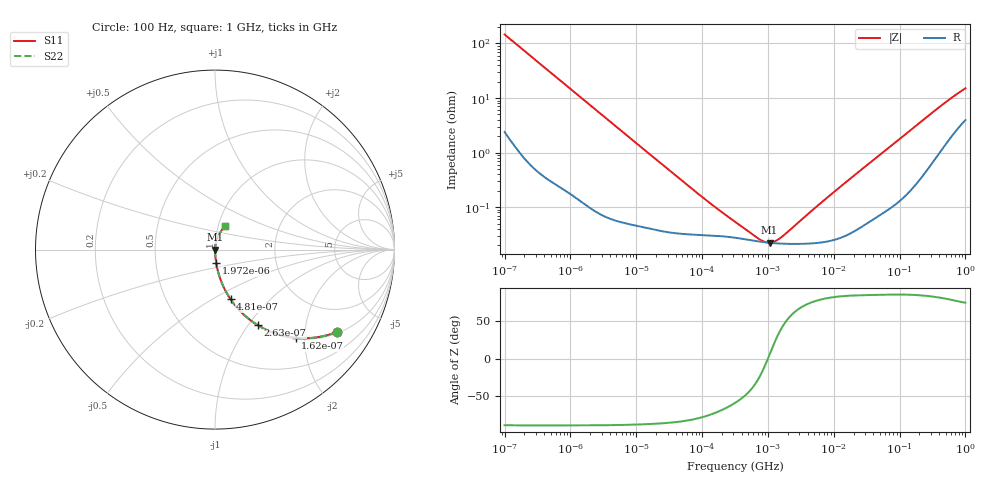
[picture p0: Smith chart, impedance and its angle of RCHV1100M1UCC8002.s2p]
! RCHV1100M1UCC8002  S-PARAMETER MODEL  (AEC-Q200 qualified)
! Model Generated by ELNA Corporation (http://www.ty-top.com)
! Version 1.0
! ELNA Control No. 240229
! Copyright (c) 2024 ELNA CO.,LTD. All Rights Reserved.
! Products Name : CONDUCTIVE POLYMER HYBRID ALUMINUM ELECTROLYTIC CAPACITORS
! Characteristics :
!  Capacitance  :  10uF  ,  Rated voltage  :  50V
!  Operating Temp. Range  :  -55 to +105 degC  ,  Endurance  :  5000hr at 105 degC
!  Dimension D  :  5mm  ,  Dimension L  :  5.8mm
! Frequency Range : 100Hz - 1GHz
! External Node Assignments :
!  1  o---| |---o  2
# MHz S RI R 50
!Freq[MHz].  S11 Real  S11 Imag  S21 Real  S21 Imag  S12 Real  S12 Imag  S22 Real  S22 Imag
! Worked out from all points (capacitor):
!   401 points, 100 Hz to 1 GHz, reference 50 ohm
!   read as one part in series: C = 10.9 uF near 108 Hz
!   lowest |Z| = 22.4 mohm at 1.059 MHz (marker M1)
!   series resonance near 1 MHz, so ESL is about 2.3 nH
!   S11 on the Smith chart (normalised r, x): 100 Hz: 1.05, -2.92; 162 Hz: 1.02, -1.80; 263 Hz: 1.01, -1.11; 481 Hz: 1.01, -0.61; 1.972 kHz: 1.00, -0.15; 1 GHz: 1.08, +0.29
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0.0001  0.6781 -0.4591  0.3219 0.4591  0.3219 0.4591  0.6781 -0.4591
0.000162  0.4485 -0.4915  0.5515 0.4915  0.5515 0.4915  0.4485 -0.4915
0.000263  0.2381 -0.421  0.7619 0.421  0.7619 0.421  0.2381 -0.421
0.000363  0.142 -0.3443  0.858 0.3443  0.858 0.3443  0.142 -0.3443
0.000481  0.087 -0.2768  0.913 0.2768  0.913 0.2768  0.087 -0.2768
0.000846  0.0311 -0.1678  0.9689 0.1678  0.9689 0.1678  0.0311 -0.1678
0.001488  0.0109 -0.0979  0.9891 0.0979  0.9891 0.0979  0.0109 -0.0979
0.001972  0.00653 -0.0743  0.9935 0.0743  0.9935 0.0743  0.00653 -0.0743
0.005188  0.00137 -0.0285  0.9986 0.0285  0.9986 0.0285  0.00137 -0.0285
0.022131  0.000417 -0.00677  0.9996 0.00677  0.9996 0.00677  0.000417 -0.00677
0.110917  0.000308 -0.00136  0.9997 0.00136  0.9997 0.00136  0.000308 -0.00136
0.316228  0.000276 -0.000465  0.9997 0.000465  0.9997 0.000465  0.000276 -0.000465
0.737055  0.000235 -0.000111  0.9998 0.000111  0.9998 0.000111  0.000235 -0.000111
0.901571  0.000227 -3.76e-05  0.9998 3.76e-05  0.9998 3.76e-05  0.000227 -3.76e-05
1.059254  0.000223 2.12e-05  0.9998 -2.12e-05  0.9998 -2.12e-05  0.000223 2.12e-05
1.295687  0.000218 9.72e-05  0.9998 -9.72e-05  0.9998 -9.72e-05  0.000218 9.72e-05
1.584893  0.000215 0.000178  0.9998 -0.000178  0.9998 -0.000178  0.000215 0.000178
4.704354  0.000218 0.000849  0.9998 -0.000849  0.9998 -0.000849  0.000218 0.000849
69.9842  0.00108 0.0124  0.9989 -0.0124  0.9989 -0.0124  0.00108 0.0124
412.0975  0.0147 0.0675  0.9853 -0.0675  0.9853 -0.0675  0.0147 0.0675
695.825  0.0343 0.1033  0.9657 -0.1033  0.9657 -0.1033  0.0343 0.1033
1000  0.0564 0.1321  0.9436 -0.1321  0.9436 -0.1321  0.0564 0.1321
